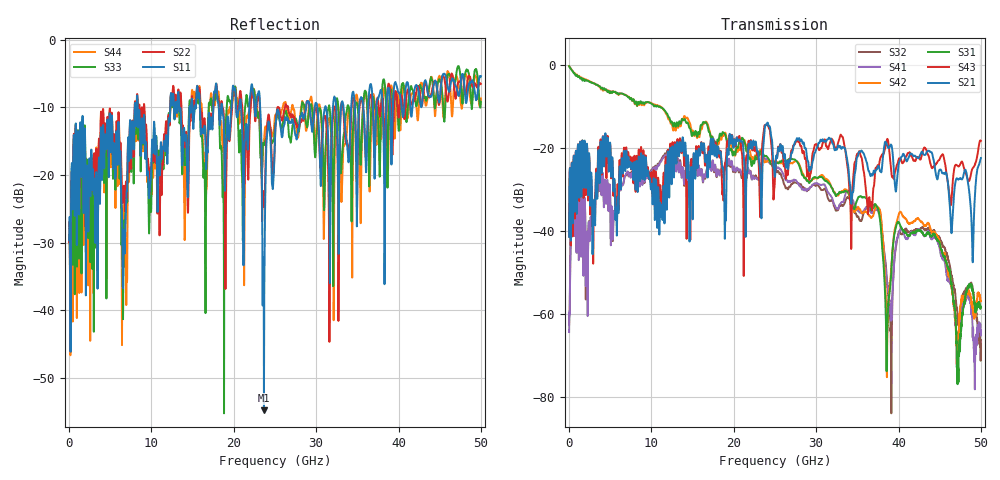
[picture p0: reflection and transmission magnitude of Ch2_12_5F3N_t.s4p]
!Agilent Technologies,N5247A,US51170199,A.09.90.13
!Agilent N5247A: A.09.90.13
!Date: Tuesday, December 08, 2015 12:46:28
!Correction: S11(Full 4 Port(1,2,3,4))
!S12(Full 4 Port(1,2,3,4))
!S13(Full 4 Port(1,2,3,4))
!S14(Full 4 Port(1,2,3,4))
!S21(Full 4 Port(1,2,3,4))
!S22(Full 4 Port(1,2,3,4))
!S23(Full 4 Port(1,2,3,4))
!S24(Full 4 Port(1,2,3,4))
!S31(Full 4 Port(1,2,3,4))
!S32(Full 4 Port(1,2,3,4))
!S33(Full 4 Port(1,2,3,4))
!S34(Full 4 Port(1,2,3,4))
!S41(Full 4 Port(1,2,3,4))
!S42(Full 4 Port(1,2,3,4))
!S43(Full 4 Port(1,2,3,4))
!S44(Full 4 Port(1,2,3,4))
!S4P File: Measurements: <S11,S12,S13,S14>,
!<S21,S22,S23,S24>,
!<S31,S32,S33,S34>,
!<S41,S42,S43,S44>:
# Hz S  dB  R 50
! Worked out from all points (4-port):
!   3201 points, 10 MHz to 50 GHz, reference 50 ohm
!   strongest paths, dB at 10 MHz, 12.51 GHz, 25 GHz, 37.5 GHz, 50 GHz:
!     S21: -41.3, -21.6, -26.9, -24.4, -22.4
!     S43: -41.3, -20.6, -27.1, -24.1, -18.3
!     S31: -0.3, -13.8, -23.6, -34.5, -58.3
!     S42: -0.3, -14.3, -23.2, -34.2, -56.9
!     S41: -64.3, -21.5, -24.3, -35.1, -65.2
!     S32: -62.5, -21.1, -25.2, -35.0, -66.2
!   lowest |S11| = -54.8 dB at 23.66 GHz (marker M1), VSWR 1.00, Z = 49.8 - j0.0286 ohm
!   |S11| at or under -10 dB: start of sweep to 7.975 GHz; 8.341 GHz to 12.29 GHz (3.947 GHz wide, 38.3 % of centre); 23.21 GHz to 28.79 GHz (5.587 GHz wide, 21.5 % of centre)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
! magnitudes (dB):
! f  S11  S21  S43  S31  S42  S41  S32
! 10 MHz  -29.7  -41.3  -41.3  -0.3  -0.3  -64.3  -62.5
! 3.915 GHz  -13.1  -20.6  -20.9  -5.6  -5.8  -30.0  -29.8
! 22.21 GHz  -6.6  -20.1  -20.3  -24.2  -22.5  -27.6  -27.6
! 23.66 GHz  -54.8  -17.7  -15.5  -21.8  -23.2  -22.3  -22.4
! 37.32 GHz  -10.1  -25.2  -24.9  -33.9  -34.2  -34.9  -34.8
! 38.61 GHz  -8.2  -19.3  -17.9  -66.0  -69.9  -53.1  -52.0
! 50 GHz  -5.4  -22.4  -18.3  -58.3  -56.9  -65.2  -66.2
